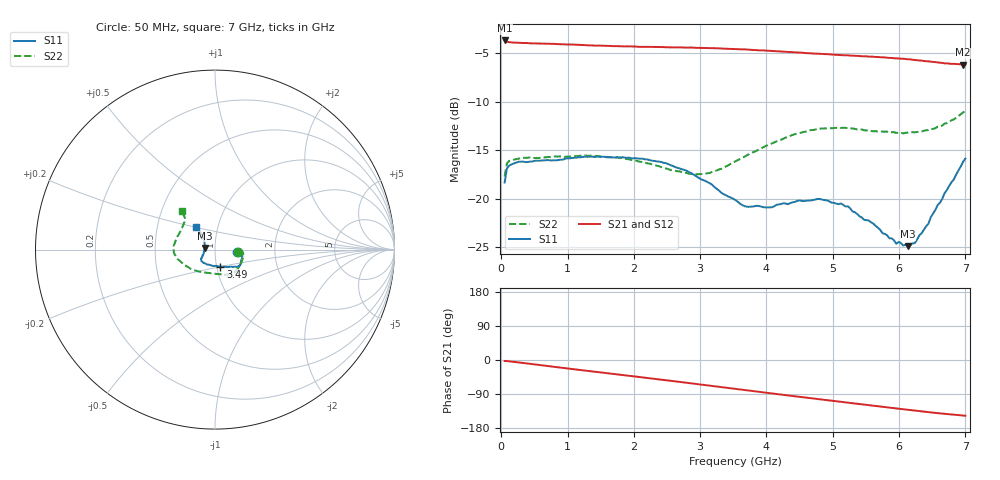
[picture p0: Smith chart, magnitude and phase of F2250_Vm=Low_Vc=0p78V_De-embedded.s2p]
! Integrated Device Technology
! Corporate Headquarters
! 6024 Silver Creek Valley Road
! San Jose, CA 95138  USA
! Phone:  1-408-284-8200
! Toll Free:  1-800-223-1366
! Webpage:  http://www.idt.com/
! Timing and RF Division
! 515 Groton Road, Suite 102
! Westford, MA 01886-6024
! Device:  F2250
! Description: Voltage Variable RF Attenuator
! Frequency:  50.0 -  6000.00 MHz
! Package:  3x3 mm Thin QFN Plastic Package: 16 pin
! Ports:  2 RF, 3 DC
!  Pin  1  = GND
!  Pin  2  = NC
!  Pin  3  = RF1  = Port 1
!  Pin  4  = NC
!  Pin  5  = GND
!  Pin  6  = GND
!  Pin  7  = GND
!  Pin  8  = GND
!  Pin  9  = NC
!  Pin 10  = RF2  = Port 2
!  Pin 11  = NC
!  Pin 12  = GND
!  Pin 13  = GND
!  Pin 14  = VCNTRL
!  Pin 15  = VDD
!  Pin 16  = VMODE
! Vcntrl:  0.780 Volts
! Vmode:  +0.000 Volts
! Vdd:  +3.30  Volts
! Current:  1.159 mA
! Data:  The device was measured on a the F2250 evaluation board which has
!  individual transmission lines to the RF pins.  Data was collected
!  using a calibrated network analyzer.  The evaluation board was
!  de-embedded using a TRL calibration technique.
!  The reference plane is the edge of the package pin.
! Misc:  SN 10
!  Action Tracker AT0258
! Date Measured:  2014-11-26
! Date:  2015-10-15  MJV
! Note:
!  Integrated Device Technology supplies this data as a sample of measured
!  data at the package pin for this product.  Your particular data for this
!  product may vary.
!  Data was taken at 25 degrees C.
!  Integrated Device Technology reserves the right to change this data at anytime.
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# GHz S dB R 50
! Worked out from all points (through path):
!   201 points, 50 MHz to 7 GHz, reference 50 ohm
!   highest |S21| = -3.70 dB at 50 MHz (marker M1); lowest = -6.2 dB at 6.965 GHz (marker M2)
!   group delay of S21, straight-line fit = 59 ps
!   lowest |S11| = -24.9 dB at 6.131 GHz (marker M3), VSWR 1.12, Z = 44.7 + j0.809 ohm
!   |S11| at or under -10 dB: start of sweep to end of sweep
!   |S22| runs from -17.7 to -10.9 dB; largest |S21 - S12| = 0.0018
!   S11 on the Smith chart (normalised r, x): 50 MHz: 1.27, -0.03; 3.49 GHz: 1.04, -0.20; 7 GHz: 0.79, +0.20
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0.05  -18.34 -6.2  -3.70 -2.5  -3.70 -2.5  -17.71 -7.1
0.08475  -16.89 -4.7  -3.83 -2.9  -3.83 -2.9  -16.36 -5.6
0.22375  -16.27 -6.9  -3.92 -5.6  -3.92 -5.6  -15.92 -9.6
1.2315  -15.70 -29.7  -4.17 -27.3  -4.19 -27.3  -15.55 -44.0
1.75275  -15.75 -35.2  -4.28 -38.1  -4.30 -38.1  -15.73 -56.0
2.37825  -16.18 -38.2  -4.37 -51.1  -4.38 -51.1  -16.65 -70.8
2.79525  -17.12 -43.8  -4.44 -60.1  -4.43 -60.1  -17.35 -87.7
3.0385  -18.07 -50.3  -4.48 -65.4  -4.48 -65.4  -17.47 -101.3
3.49025  -19.97 -72.3  -4.58 -75.4  -4.58 -75.4  -16.28 -127.8
3.525  -20.12 -73.8  -4.58 -76.1  -4.59 -76.1  -16.17 -129.6
3.69875  -20.82 -86.2  -4.63 -80.0  -4.64 -80.0  -15.55 -138.1
3.97675  -20.90 -104.2  -4.73 -86.0  -4.75 -86.0  -14.61 -150.8
4.7065  -20.14 -137.7  -5.04 -101.7  -5.04 -101.7  -12.92 -173.4
5.22775  -20.78 -148.0  -5.23 -112.6  -5.24 -112.6  -12.72 174.9
5.85325  -24.09 -166.8  -5.49 -125.6  -5.49 -125.6  -13.16 159.1
5.9575  -24.65 -174.1  -5.54 -127.8  -5.54 -127.8  -13.22 156.1
6.13125  -24.89 170.9  -5.63 -131.4  -5.63 -131.4  -13.19 150.2
6.2355  -24.58 159.1  -5.70 -133.5  -5.70 -133.6  -13.17 146.8
6.444  -22.56 142.5  -5.84 -137.7  -5.85 -137.7  -12.92 140.1
6.722  -19.09 131.1  -6.06 -142.5  -6.06 -142.6  -12.21 133.3
6.96525  -16.20 130.1  -6.18 -146.5  -6.17 -146.6  -11.11 131.6
7  -15.86 129.8  -6.18 -147.0  -6.17 -147.1  -10.95 131.0
